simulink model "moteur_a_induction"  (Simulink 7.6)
settings: Solver=ode15s  StartTime=0.0  StopTime=20.0  RelTol=1e-3
InitFcn:
  | clear all
  | close all
  | delete *.mat
  | clc
StopFcn:
  | load mot_ind_pos_vit.mat
  | plotyy(x(1,:),x(2,:), x(1,:),x(3,:))
  | grid
  | title('Moteur à induction - Position et Vitesse')
  | xlabel('temps')
libraries: nesl_utility x7, fl_lib x6, elec_lib x1

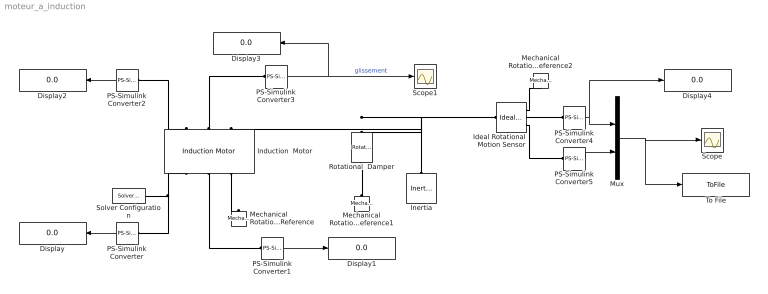
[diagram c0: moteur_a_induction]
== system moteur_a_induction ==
  Display{,1..4} (5 alike) : Display
  Ideal Rotational Motion Sensor : fl_lib/Mechanical/Mechanical Sensors/Ideal Rotational Motion Sensor  DialogController=NetworkEngine.DynNeDlgSource  SystemSampleTime=-1  offset=0 rad  w_Log=off  t_Log=off  phi_Log=off  LocalVarNames=|w|t|phi  LocalVarDescs=|w|t|phi  LocalVarLogging=[0 0 0]
  Induction  Motor : elec_lib/Actuators & Drivers/Rotational Actuators/Induction Motor  DialogController=NetworkEngine.DynNeDlgSource  SystemSampleTime=-1  param=1  R1=1 Ohm  R2=1 Ohm  L1=0.02 H  L2=0.02 H  Lm=0.5 H  P_rated=825 W  w_mech=3.5e+03 rpm  v_rated=200 V  w_rated=60 Hz  i_rated=2.7 A  paramL=1  i_start=7.5 A  T_max=3.3 N*m  paramR1=1  E=95  pf=0.93  R1m=1 Ohm  V=200 V  w=60 Hz  p=1  n=3  paramLoad=1  J=0.001 kg*m^2  lam=1e-04 N*m/(rad/s)  speed0=0 rpm  LocalVarLogging=[]
  Inertia : fl_lib/Mechanical/Rotational Elements/Inertia  DialogController=NetworkEngine.DynNeDlgSource  SystemSampleTime=-1  inertia=0.01 kg*m^2  initial_velocity=0 rad/s  t_Log=off  LocalVarNames=|t  LocalVarDescs=|t  LocalVarLogging=0
  Mechanical Rotational Reference : fl_lib/Mechanical/Rotational Elements/Mechanical Rotational Reference  DialogController=NetworkEngine.DynNeDlgSource  SystemSampleTime=-1  t_Log=off  LocalVarNames=|t  LocalVarDescs=|t  LocalVarLogging=0
  Mechanical Rotational Reference1 : fl_lib/Mechanical/Rotational Elements/Mechanical Rotational Reference  DialogController=NetworkEngine.DynNeDlgSource  SystemSampleTime=-1  t_Log=off  LocalVarNames=|t  LocalVarDescs=|t  LocalVarLogging=0
  Mechanical Rotational Reference2 : fl_lib/Mechanical/Rotational Elements/Mechanical Rotational Reference  DialogController=NetworkEngine.DynNeDlgSource  SystemSampleTime=-1  t_Log=off  LocalVarNames=|t  LocalVarDescs=|t  LocalVarLogging=0
  Mux : Mux  Inputs=2
  PS-Simulink Converter{,1..5} (6 alike) : nesl_utility/PS-Simulink Converter  DialogController=NetworkEngine.DynNeUtilDlgSource  SystemSampleTime=-1  PhysicalDomain=network_engine_domain  LeftPortType=input  RightPortType=output  SubClassName=ps_output  Unit=1  AffineConversion=off
  Rotational  Damper : fl_lib/Mechanical/Rotational Elements/Rotational Damper  DialogController=NetworkEngine.DynNeDlgSource  SystemSampleTime=-1  D=0.001 N*m/(rad/s)  t_Log=off  w_Log=off  LocalVarNames=|t|w  LocalVarDescs=|t|w  LocalVarLogging=[0 0]
  Scope : Scope
  Scope1 : Scope
  Solver Configuration : nesl_utility/Solver Configuration  DialogController=NetworkEngine.DynNeUtilDlgSource  SystemSampleTime=-1  PhysicalDomain=network_engine_domain  LeftPortType=input  RightPortType=generic  SubClassName=solver  Accelerate=off  Profile=off  ResidualTolerance=1e-9  MaxNonlinIter=12  MaxModeIter=2  DoFixedCost=off  UseLocalSampling=off  DoDC=off  LinearAlgebra=Sparse  LocalSolverSampleTime=.001  LocalSolverChoice=NE_BACKWARD_EULER_ADVANCER  UseLocalSolver=off
  To File : ToFile  Filename=mot_ind_pos_vit  MatrixName=x
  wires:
  PS-Simulink Converter/1 -> Display/1
  PS-Simulink Converter1/1 -> Display1/1
  PS-Simulink Converter2/1 -> Display2/1
  PS-Simulink Converter3/1 -> Display3/1, Scope1/1  "glissement"
  PS-Simulink Converter4/1 -> Mux/1, Display4/1
  PS-Simulink Converter5/1 -> Mux/2
  Mux/1 -> Scope/1, To File/1
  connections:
  PS-Simulink Converter/LConn1 -- Induction  Motor/RConn1 -- Solver Configuration/RConn1
  Induction  Motor/RConn2 -- PS-Simulink Converter1/LConn1
  PS-Simulink Converter2/LConn1 -- Induction  Motor/LConn1
  Induction  Motor/RConn3 -- Mechanical Rotational Reference/LConn1
  Rotational  Damper/LConn1 -- Induction  Motor/LConn3 -- Ideal Rotational Motion Sensor/LConn1 -- Inertia/LConn1
  Rotational  Damper/RConn1 -- Mechanical Rotational Reference1/LConn1
  Ideal Rotational Motion Sensor/RConn1 -- Mechanical Rotational Reference2/LConn1
  Ideal Rotational Motion Sensor/RConn2 -- PS-Simulink Converter4/LConn1
  Ideal Rotational Motion Sensor/RConn3 -- PS-Simulink Converter5/LConn1
  Induction  Motor/LConn2 -- PS-Simulink Converter3/LConn1
